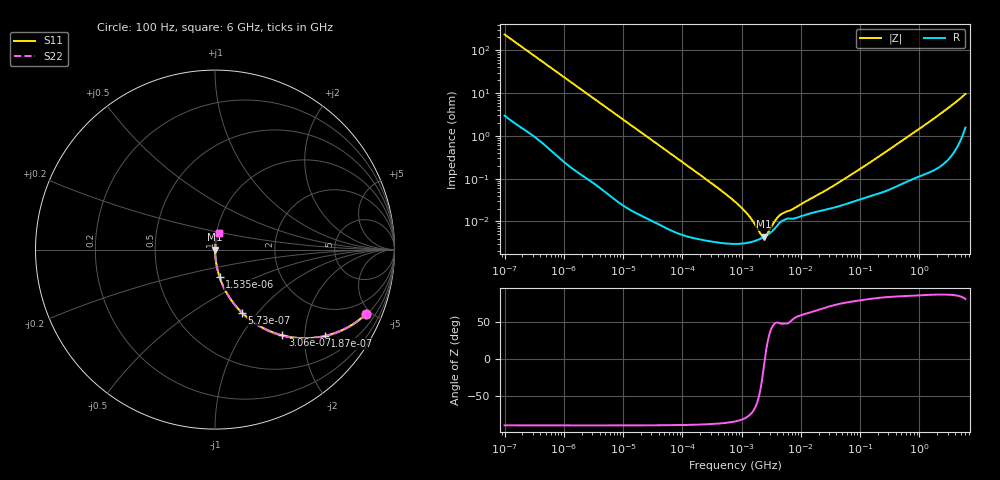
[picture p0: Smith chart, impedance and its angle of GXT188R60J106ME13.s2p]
!Murata Part Number: GXT188R60J106ME13
!These Parameters are Measured in Series Mode Connection
!Data Generated on Jan 08, 2026
!  o--ll--o
!Port1  Port2
!  o------o
!Operation Temp=25[degC], DC Bias Voltage=0[V]
!Freq. Start=100[Hz] Stop=6[GHz] 401[Steps]
# Hz S RI R 50
!Freq.(Hz) S11(Real) S11(Imag) S21(Real) S21(Imag) S12(Real) S12(Imag) S22(Real) S22(Imag)
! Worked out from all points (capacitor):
!   401 points, 100 Hz to 6 GHz, reference 50 ohm
!   read as one part in series: C = 6.76 uF near 109 Hz
!   lowest |Z| = 4.4 mohm at 2.373 MHz (marker M1)
!   series resonance near 2.474 MHz, so ESL is about 610 pH
!   S11 on the Smith chart (normalised r, x): 100 Hz: 1.06, -4.69; 187 Hz: 1.03, -2.52; 306 Hz: 1.02, -1.55; 573 Hz: 1.01, -0.83; 1.535 kHz: 1.00, -0.31; 6 GHz: 1.03, +0.19
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100  0.8432 -0.3573  0.1568 0.3573  0.1568 0.3573  0.8432 -0.3573
131  0.7609 -0.4204  0.2391 0.4204  0.2391 0.4204  0.7609 -0.4204
187  0.612 -0.481  0.388 0.481  0.388 0.481  0.612 -0.481
306  0.3756 -0.4779  0.6244 0.4779  0.6244 0.4779  0.3756 -0.4779
573  0.15 -0.3513  0.85 0.3513  0.85 0.3513  0.15 -0.3513
897  0.0684 -0.2473  0.9316 0.2473  0.9316 0.2473  0.0684 -0.2473
1535  0.0252 -0.1518  0.9748 0.1518  0.9748 0.1518  0.0252 -0.1518
2008  0.0152 -0.1175  0.9848 0.1175  0.9848 0.1175  0.0152 -0.1175
6433  0.00178 -0.0375  0.9982 0.0375  0.9982 0.0375  0.00178 -0.0375
40335  0.000122 -0.00605  0.9999 0.00605  0.9999 0.00605  0.000122 -0.00605
330837  3.4e-05 -0.000734  1 0.000734  1 0.000734  3.4e-05 -0.000734
774597  3e-05 -0.000289  1 0.000289  1 0.000289  3e-05 -0.000289
1585629  3.42e-05 -9.14e-05  1 9.14e-05  1 9.14e-05  3.42e-05 -9.14e-05
2372521  4.32e-05 -8.2e-06  1 8.2e-06  1 8.2e-06  4.32e-05 -8.2e-06
3549919  6.6e-05 7.05e-05  0.9999 -7.05e-05  0.9999 -7.05e-05  6.6e-05 7.05e-05
4856642  0.000103 0.000112  0.9999 -0.000112  0.9999 -0.000112  0.000103 0.000112
7266822  0.000116 0.000155  0.9999 -0.000155  0.9999 -0.000155  0.000116 0.000155
1.555665e7  0.000159 0.000317  0.9998 -0.000317  0.9998 -0.000317  0.000159 0.000317
4.983056e7  0.00024 0.000881  0.9998 -0.000881  0.9998 -0.000881  0.00024 0.000881
3.124326e8  0.000579 0.00481  0.9994 -0.00481  0.9994 -0.00481  0.000579 0.00481
1.95892e9  0.00249 0.0281  0.9975 -0.0281  0.9975 -0.0281  0.00249 0.0281
6e9  0.0238 0.0906  0.9762 -0.0906  0.9762 -0.0906  0.0238 0.0906
